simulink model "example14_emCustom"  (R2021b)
settings: Solver=FixedStepAuto  StartTime=0  StopTime=inf  FixedStep=0.5  RelTol=1e-3  EnableMultiTasking=on
undefined symbols (not defined in the file or in its folder): based, classic, dsPic33, MCC, Microchip, PIC24, U1, U2, Y1, Y2
libraries: embeddedCreatorLib x6, emMBSlaveLib x1

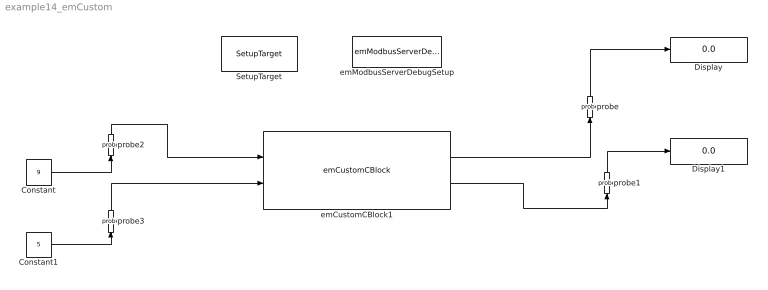
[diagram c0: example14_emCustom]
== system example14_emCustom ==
  Constant : Constant  Value=9  OutDataTypeStr=int16
  Constant1 : Constant  Value=5  OutDataTypeStr=int16
  Display : Display
  Display1 : Display
  SetupTarget : embeddedCreatorLib/SetupTarget  Tag=SetupTarget  Priority=0  c_platform=Microchip PIC24/dsPic33 based on MCC classic  c_debug=on
  emCustomCBlock1 : embeddedCreatorLib/emCustomCBlock  Tag=emCustomBlock  c_InputDataName=[U1 U2]  c_InputDataType=[int16 int16]  c_OutputDataName=[Y1 Y2]  c_OutputDataType=[int16 int16]  c_InputDataQty="[1  1]"  c_InputType="[4  4]"  c_OutputDataQty="[1  1]"  c_OutputType="[4  4]"  c_sampleTime=-1  c_blockname=emCustomCBlock1
  emModbusServerDebugSetup : emMBSlaveLib/emModbusServerDebugSetup  Tag=emModbusSlaveSetup  c_objID=0  c_uartNo=2  c_baudrate=19200  c_serverID=1  c_baudrate4PC=19200  c_forceLongerSpace=on  c_holdingRegsQTY=0  c_minHoldingAddr=789  c_inputRegsQTY=0  c_minInputRegAddr=20  c_coilRegsQTY=0  c_minCoilAddr=30  c_discreteRegsQTY=0  c_minDiscreteAddr=40  c_enableDebug=on  c_breakpointMaxQTY=0  c_probeMaxWordQTY=100  c_emWaitQTY=0  g_COMPortNo=COM5  c_Name_method=By physical port name and bit number  c_PortName=B  c_BitNo=11  c_TxEnable485="\"LATBbits.LATB11\""  c_TxEnable485Polarity=on
  probe : embeddedCreatorLib/probe  Tag=emProbe  c_ObjID=2  c_serverID=1  c_UartNo=2  c_StartAddr=4  c_ConstantDataSource=off
  probe1 : embeddedCreatorLib/probe  Tag=emProbe  c_ObjID=3  c_serverID=1  c_UartNo=2  c_StartAddr=5  c_ConstantDataSource=off
  probe2 : embeddedCreatorLib/probe  Tag=emProbe  c_ObjID=0  c_serverID=1  c_UartNo=2  c_StartAddr=2  c_ConstantDataSource=on
  probe3 : embeddedCreatorLib/probe  Tag=emProbe  c_ObjID=1  c_serverID=1  c_UartNo=2  c_StartAddr=3  c_ConstantDataSource=on
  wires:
  emCustomCBlock1/1 -> probe/1
  probe/1 -> Display/1
  probe1/1 -> Display1/1
  emCustomCBlock1/2 -> probe1/1
  Constant/1 -> probe2/1
  probe2/1 -> emCustomCBlock1/1
  Constant1/1 -> probe3/1
  probe3/1 -> emCustomCBlock1/2
